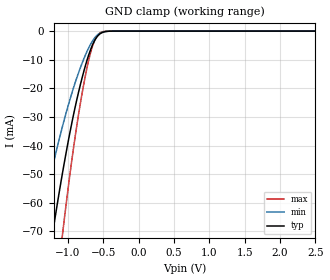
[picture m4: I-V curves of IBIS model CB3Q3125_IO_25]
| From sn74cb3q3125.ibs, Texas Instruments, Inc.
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[Model]   CB3Q3125_IO_25
Model_type  Terminator
| variable   typ   min   max
C_comp   4.00pF   3.31pF   4.28pF
| C_tri-state   4.00pF   3.31pF   4.28pF
[Temperature Range]   40   100   -40
| Ambient temperature   25   85   -40
[Voltage range]   2.5   2.3   2.7
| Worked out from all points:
|   GND clamp passes 1 mA (typ) near -0.55 V on its own axis
[GND Clamp]
| CB3Q3125_IO_25
|   Voltage   I(typ)   I(min)   I(max)
-5.5V     -1.051A    -807.9mA   -1.307A
-1.43V    -107mA     -72.03mA   -152.9mA
-1.405V   -102.5mA   -68.95mA   -146.7mA
-1.22V    -71.16mA   -47.68mA   -102.4mA
-1.2V     -67.99mA   -45.55mA   -97.84mA
-1.08V    -49.95mA   -33.53mA   -71.58mA
-1.06V    -47.13mA   -31.66mA   -67.42mA
-895mV    -26.2mA    -17.81mA   -36.32mA
-775mV    -13.99mA   -9.653mA   -18.32mA
-655mV    -4.955mA   -3.544mA   -5.396mA
-550mV    -1.009mA   -786.7uA   -674.3uA
2.5V      147.2pA    716.2pA    14.5pA
